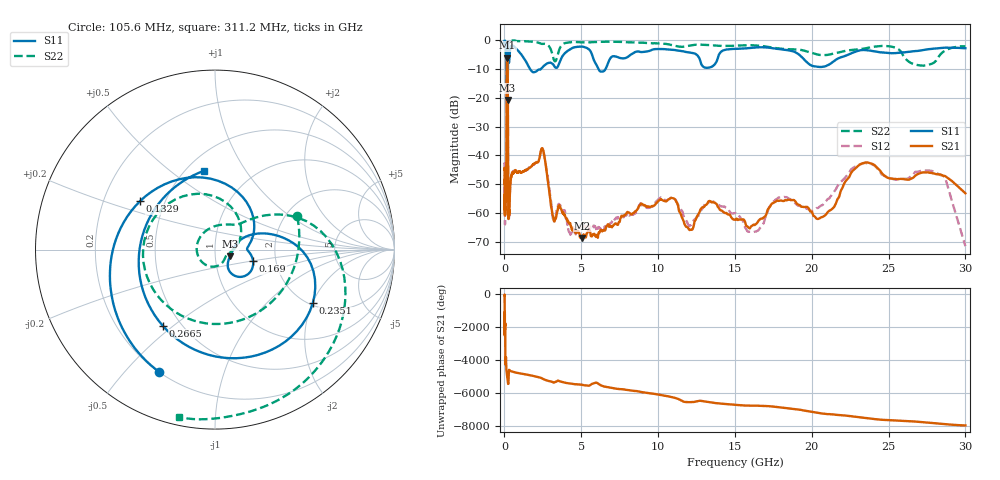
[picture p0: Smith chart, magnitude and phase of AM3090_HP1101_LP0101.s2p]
! Date/Time: Thu, Feb 28, 2019 2:07 PM
! Network Analyzer: Agilent Technologies E8364B Rev: A.07.50.67
! Sweep from 0.010 to 30.000 GHz, 1601 Points, Sweep Type: LOG
! Power Supply: 5.022 V, 0.002 A
# Hz S DB R 50
!freq MagS11 AngS11 MagS21 AngS21 MagS12 AngS12 MagS22 AngS22
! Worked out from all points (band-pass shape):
!   1601 points, 10 MHz to 30 GHz, reference 50 ohm
!   highest |S21| = -6.16 dB at 175.9 MHz (marker M1); lowest = -68.6 dB at 5.077 GHz (marker M2)
!   |S21| within 3 dB of the highest: 150.1 MHz to 207.6 MHz (57.5 MHz wide, 32.2 % of centre)
!   lowest |S11| = -20.8 dB at 198.3 MHz (marker M3), VSWR 1.20, Z = 58.9 - j4.48 ohm
!   |S11| at or under -10 dB: 144.1 MHz to 218.6 MHz (74.52 MHz wide, 41.1 % of centre); 1.657 GHz to 2.379 GHz (721.5 MHz wide, 35.7 % of centre); 6.111 GHz to 6.584 GHz (473.2 MHz wide, 7.46 % of centre)
!   |S22| runs from -23.0 to -0.1 dB; largest |S21 - S12| = 0.013
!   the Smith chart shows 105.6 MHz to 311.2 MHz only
!   S11 on the Smith chart (normalised r, x): 105.6 MHz: 0.20, -0.62; 132.9 MHz: 0.36, +0.26; 169 MHz: 1.52, -0.20; 235.1 MHz: 2.07, -2.02; 266.5 MHz: 0.40, -0.46; 311.2 MHz: 0.61, +0.67
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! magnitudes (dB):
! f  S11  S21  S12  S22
! 10 MHz  -0.3  -45.0  -43.0  -0.5
! 38.04 MHz  -0.4  -56.7  -57.6  -1.2
! 105.6 MHz  -2.5  -55.3  -55.7  -6.1
! 117.9 MHz  -3.6  -52.3  -51.5  -7.5
! 132.9 MHz  -6.1  -28.6  -28.5  -8.0
! 144.7 MHz  -10.3  -12.8  -12.7  -13.0
! 169 MHz  -13.1  -6.2  -6.2  -21.0
! 175.9 MHz  -12.7  -6.2  -6.1  -20.1
! 198.3 MHz  -20.8  -7.3  -7.3  -17.3
! 235.1 MHz  -4.1  -40.0  -40.5  -2.6
! 266.5 MHz  -5.8  -61.0  -60.9  -0.8
! 311.2 MHz  -7.1  -60.3  -60.8  -0.4
! 550.5 MHz  -2.0  -46.3  -45.6  -0.2
! 2.084 GHz  -10.8  -42.5  -42.3  -0.7
! 2.495 GHz  -9.4  -37.8  -37.7  -1.3
! 5.077 GHz  -2.3  -68.6  -63.2  -0.8
! 7.926 GHz  -6.1  -60.1  -60.9  -0.8
! 16.21 GHz  -2.7  -64.0  -66.7  -1.8
! 20.82 GHz  -9.2  -61.0  -56.4  -5.2
! 23.48 GHz  -3.5  -42.5  -42.7  -2.9
! 27.83 GHz  -3.1  -46.2  -45.4  -8.2
! 30 GHz  -2.8  -53.2  -71.5  -2.2
